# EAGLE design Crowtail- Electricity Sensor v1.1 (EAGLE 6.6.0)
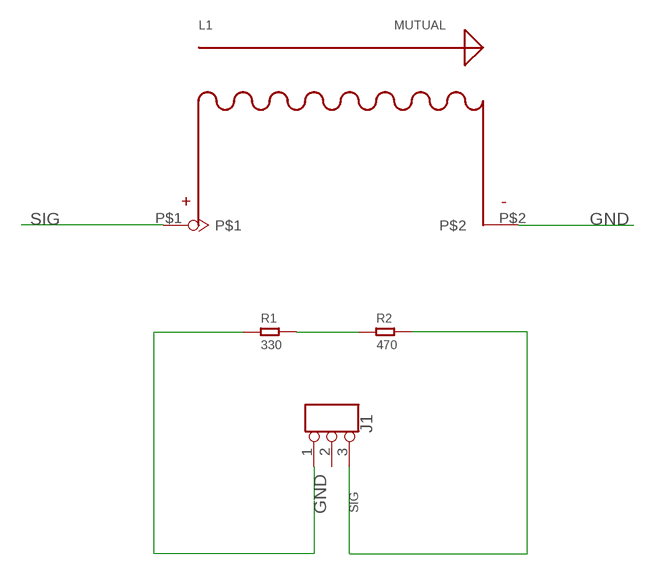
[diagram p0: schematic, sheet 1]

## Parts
J1  TINKER_3P_DIP  [3P_2.0_DIP]
L1  MUTUAL  [MUTUAL]
R1  330  R-0603  [R0603]
R2  470  R-0603  [R0603]

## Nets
GND: J1.1 L1.P$2 R1.1
N$2: R1.2 R2.1
SIG: J1.3 L1.P$1 R2.2
Unconnected: J1.2

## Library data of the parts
J1 = Connector:TINKER_3P_DIP
L1 = AnlogDevice:MUTUAL
R1 R2 = Discrete:R*

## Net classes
1 power: width 0.61 mm, drill 0.406 mm, clearance 0.203 mm
2 gnd: width 0.305 mm, drill 0.559 mm, clearance 0.254 mm
3 usbvcc: width 0.508 mm, drill 0.61 mm, clearance 0.254 mm

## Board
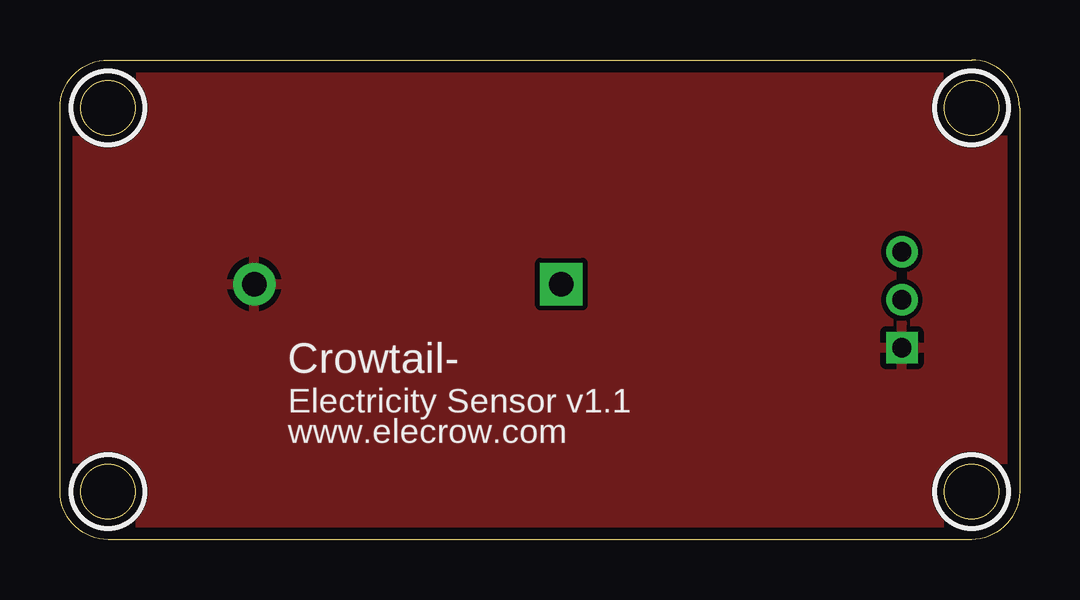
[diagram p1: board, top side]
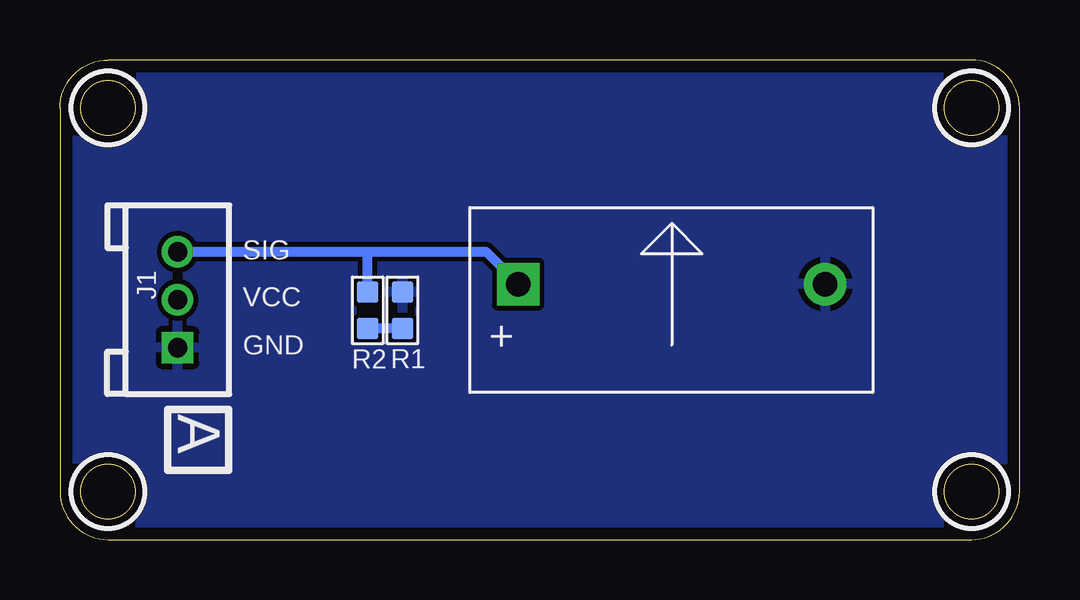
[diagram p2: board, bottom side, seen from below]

Size 40 x 20 mm. Coordinates in mm from the lower left corner, seen from the top.
Outline: 40,18 40,2 arc-90 38,0 2,0 arc-90 0,2 0,18 arc-90 2,20 38,20 arc-90 40,18
Outline: circle at 38,18 radius 1.14
Outline: circle at 38,2 radius 1.14
Outline: circle at 2,18 radius 1.14
Outline: circle at 2,2 radius 1.14
Copper layers (1*16): Top 0.035mm / dielectric 1.5mm / Bottom 0.035mm
Design rules: minimum track width 10mil, minimum drill 12mil, track to track 8mil, track to pad 8mil, pad to pad 8mil, via to via 8mil, smd to smd 8mil, copper to edge 20mil, drill to drill 8mil, minimum pad ring 10mil, minimum via ring 8mil, stop-mask expansion 2mil, vias tented up to drill 100mil, thermal gap 10mil
tRestrict: area 36.5,16.5 to 39.5,19.5; area 36.5,0.5 to 39.5,3.5; area 0.5,16.5 to 3.5,19.5; area 0.5,0.5 to 3.5,3.5
bRestrict: area 36.5,16.5 to 39.5,19.5; area 36.5,0.5 to 39.5,3.5; area 0.5,16.5 to 3.5,19.5; area 0.5,0.5 to 3.5,3.5

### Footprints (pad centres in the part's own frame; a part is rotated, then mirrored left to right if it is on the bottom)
3P_2.0_DIP = drill 0.8 pad 1.27 square: 1 -2,0 | drill 0.8 pad 1.27: 2 0,0; 3 2,0
MUTUAL = drill 1.016 pad 1.778 square: P$1 -6.4,0 | drill 1.016 pad 1.778: P$2 6.4,0
R0603 = smd 0.889 x 0.889: 1 -0.762,0; 2 0.762,0

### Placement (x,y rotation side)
J1  35.1,10 90 bottom
L1  14.5,10.65 0 bottom
R1  25.72,9.56 270 bottom
R2  27.18,9.56 90 bottom

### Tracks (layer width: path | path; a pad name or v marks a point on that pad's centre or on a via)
GND
  pour Bottom: 40,20.32 -0.64,20.32 -0.64,0 40,0
  pour Top: 40,20.32 -0.64,20.32 -0.64,0 40,0
N$2
  Bottom 0.406: R1.2 R2.1
SIG
  Bottom 0.406: J1.3 27.2,12 | 27.2,12 22.25,12 L1.P$1 | R2.2 27.18,11.98 27.2,12

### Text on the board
tPlace: Crowtail- | Electricity Sensor v1.1 | www.elecrow.com
bPlace: A
bNames: SIG | VCC | GND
